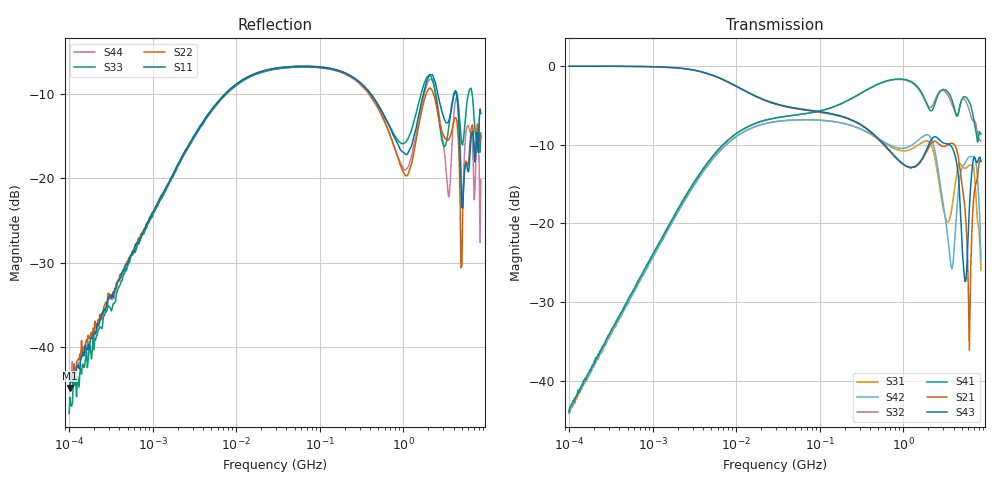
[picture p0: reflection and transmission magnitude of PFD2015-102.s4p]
# MHz S MA R 50
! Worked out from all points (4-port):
!   498 points, 100 kHz to 8.5 GHz, reference 50 ohm
!   strongest paths, dB at 100 kHz, 1.698 MHz, 29.49 MHz, 500.7 MHz, 8.5 GHz:
!     S43: -0.1, -0.2, -4.8, -9.2, -12.1
!     S21: 0.0, -0.2, -4.9, -9.3, -12.2
!     S41: -43.9, -19.6, -6.6, -2.3, -8.7
!     S32: -43.8, -19.6, -6.6, -2.3, -9.6
!     S42: -44.2, -20.0, -7.1, -9.2, -24.7
!     S31: -44.1, -19.9, -7.1, -9.3, -26.0
!   lowest |S11| = -44.9 dB at 102.3 kHz (marker M1), VSWR 1.01, Z = 49.9 + j0.563 ohm
!   |S11| at or under -10 dB: 413.5 MHz to 1.74 GHz (1.326 GHz wide, 123 % of centre); 2.6 GHz to 4.064 GHz (1.464 GHz wide, 43.9 % of centre); 4.324 GHz to end of sweep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
0.1  0.005752 100.9  0.9946 -0.4  0.006247 -93.5  0.006352 89.5
     0.9946 -0.4  0.006496 93.9  0.006446 87.8  0.0062 -91.6
     0.006247 -93.5  0.006446 87.8  0.004023 62.7  0.9934 -0.3
     0.006352 89.5  0.0062 -91.6  0.9934 -0.3  0.006664 89.7
0.1023101  0.005684 97.3  0.9941 -0.4  0.006293 -93.6  0.006771 86.2
           0.9941 -0.4  0.006898 99.4  0.006749 87.2  0.00648 -91.7
           0.006293 -93.6  0.006749 87.2  0.005004 75.3  0.9937 -0.3
           0.006771 86.2  0.00648 -91.7  0.9937 -0.3  0.005712 82.5
17.04623  0.4211 20.9  0.6388 -21.0  0.4115 -160.1  0.4306 24.7
          0.6388 -21.0  0.4208 20.6  0.431 24.7  0.411 -160.3
          0.4115 -160.1  0.431 24.7  0.4153 21.2  0.6429 -20.9
          0.4306 24.7  0.411 -160.3  0.6429 -20.9  0.4154 20.9
389.4413  0.3285 -82.6  0.3861 -100.1  0.3722 78.9  0.7165 -36.3
          0.3861 -100.1  0.3208 -87.7  0.7149 -36.4  0.3738 74.2
          0.3722 78.9  0.7149 -36.4  0.3265 -82.2  0.3895 -100.6
          0.7165 -36.3  0.3738 74.2  0.3895 -100.6  0.3165 -87.7
1277.015  0.1601 -162.9  0.2258 83.9  0.2979 -94.8  0.7871 -174.4
          0.2258 83.9  0.1255 -158.7  0.7769 -174.2  0.3147 -100.7
          0.2979 -94.8  0.7769 -174.2  0.1993 -161.2  0.2273 81.0
          0.7871 -174.4  0.3147 -100.7  0.2273 81.0  0.1403 -161.6
2776.003  0.2728 -33.6  0.3132 97.3  0.1601 -60.3  0.6892 2.3
          0.3132 97.3  0.2059 -23.1  0.691 -0.2  0.1766 -47.1
          0.1601 -60.3  0.691 -0.2  0.1956 -21.3  0.3345 92.5
          0.6892 2.3  0.1766 -47.1  0.3345 92.5  0.2147 -53.7
8500  0.2434 -34.7  0.2464 29.4  0.05037 6.6  0.3682 -35.9
      0.2464 29.4  0.1795 -44.0  0.3323 -31.8  0.058 -52.0
      0.05037 6.6  0.3323 -31.8  0.1861 -17.6  0.2474 17.3
      0.3682 -35.9  0.058 -52.0  0.2474 17.3  0.09864 10.5
